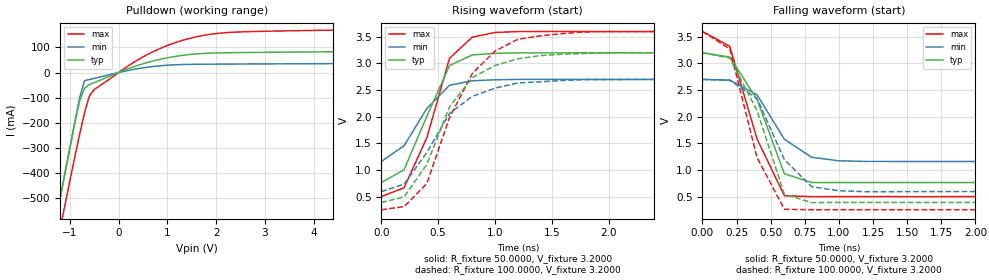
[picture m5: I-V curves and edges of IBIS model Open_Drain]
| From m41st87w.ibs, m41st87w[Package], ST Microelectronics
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|   Model Open_Drain
[Model]   Open_Drain
Model_type   Open_drain
Polarity   Inverting
Vmeas =   1.5000V
Cref =  50.0000pF
Rref =   0.6450k
Vref =   1.7500V
C_comp   6.3700pF   6.5600pF   6.1200pF
[Temperature Range]   27.0000   85.0000   -40.0000
[Voltage Range]   3.2000V   2.7000V   3.6000V
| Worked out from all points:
|   slope of the pulldown table from 0 to 0.48 V, typ, clamps not added: 14.3 ohm
|   rising waveform, R_fixture 50.0000, V_fixture 3.2000: 20-80 % time 299ps typ, 305ps min, 288ps max; typ from 0.763 V to 3.2 V
|   rising waveform, R_fixture 100.0000, V_fixture 3.2000: 20-80 % time 414ps typ, 440ps min, 427ps max; typ from 0.389 V to 3.2 V
|   falling waveform, R_fixture 50.0000, V_fixture 3.2000: 20-80 % time 251ps typ, 260ps min, 248ps max; typ from 3.2 V to 0.763 V
|   falling waveform, R_fixture 100.0000, V_fixture 3.2000: 20-80 % time 254ps typ, 260ps min, 230ps max; typ from 3.2 V to 0.389 V
[Pulldown]
| voltage   I(typ)   I(min)   I(max)
-3.2V     -2.5A      -2.5A      -2.591A
-1.4V     -700mA     -700mA     -815.7mA
-1V       -300mA     -300mA     -430.8mA
-800mV    -114.1mA   -100mA     -246.1mA
-700mV    -62.82mA   -32.69mA   -160.6mA
-600mV    -47.72mA   -27.8mA    -93.29mA
-500mV    -39.9mA    -23.29mA   -67.68mA
100mV     7.895mA    4.371mA    13.86mA
800mV     50.46mA    25.78mA    91.44mA
1.5V      72.58mA    32.65mA    138.2mA
2.5V      79.48mA    33.9mA     161.8mA
6.4V      86.87mA    37.52mA    176.6mA
[Ramp]
| variable   typ   min   max
dV/dt_r   1.8814/2.6846n   1.5630/2.8045n   2.1342/2.5575n
dV/dt_f   1.8837/0.1927n   1.5646/0.2534n   2.1364/0.1595n
R_load = 0.6450k
[Rising Waveform]
R_fixture = 50.0000
V_fixture = 3.2000
V_fixture_min = 2.7000
V_fixture_max = 3.6000
| time   V(typ)   V(min)   V(max)
0s        762.9mV    1.158V     498.2mV
200ps     1.003V     1.453V     665.5mV
400ps     2.006V     2.154V     1.602V
600ps     2.962V     2.591V     3.097V
800ps     3.16V      2.675V     3.496V
1ns       3.19V      2.694V     3.583V
1.4ns     3.2V       2.701V     3.6V
10ns      3.2V       2.7V       3.6V
[Rising Waveform]
R_fixture = 100.0000
V_fixture = 3.2000
V_fixture_min = 2.7000
V_fixture_max = 3.6000
| time   V(typ)   V(min)   V(max)
0s        389mV      592.5mV    251.5mV
200ps     492.6mV    732.6mV    310.4mV
400ps     1.101V     1.326V     741.3mV
600ps     2.186V     2.061V     1.985V
800ps     2.735V     2.382V     2.811V
1ns       2.962V     2.537V     3.233V
1.2ns     3.088V     2.635V     3.454V
1.4ns     3.148V     2.655V     3.52V
1.8ns     3.188V     2.698V     3.596V
10ns      3.2V       2.7V       3.6V
[Falling Waveform]
R_fixture = 50.0000
V_fixture = 3.2000
V_fixture_min = 2.7000
V_fixture_max = 3.6000
| time   V(typ)   V(min)   V(max)
0s        3.2V       2.7V       3.6V
200ps     3.12V      2.686V     3.323V
400ps     2.325V     2.411V     1.583V
600ps     928.7mV    1.576V     516.2mV
800ps     762.7mV    1.237V     497.2mV
1ns       762.9mV    1.171V     498.8mV
1.2ns     762.8mV    1.159V     498.4mV
10ns      762.9mV    1.158V     497.6mV
[Falling Waveform]
R_fixture = 100.0000
V_fixture = 3.2000
V_fixture_min = 2.7000
V_fixture_max = 3.6000
| time   V(typ)   V(min)   V(max)
0s        3.2V       2.7V       3.6V
200ps     3.102V     2.684V     3.274V
400ps     2.114V     2.342V     1.233V
600ps     544.8mV    1.194V     260.3mV
800ps     385.4mV    684.9mV    251.6mV
1ns       389.1mV    609.3mV    251.5mV
1.2ns     389.6mV    590.1mV    251.5mV
10ns      389.2mV    592.9mV    251.5mV
